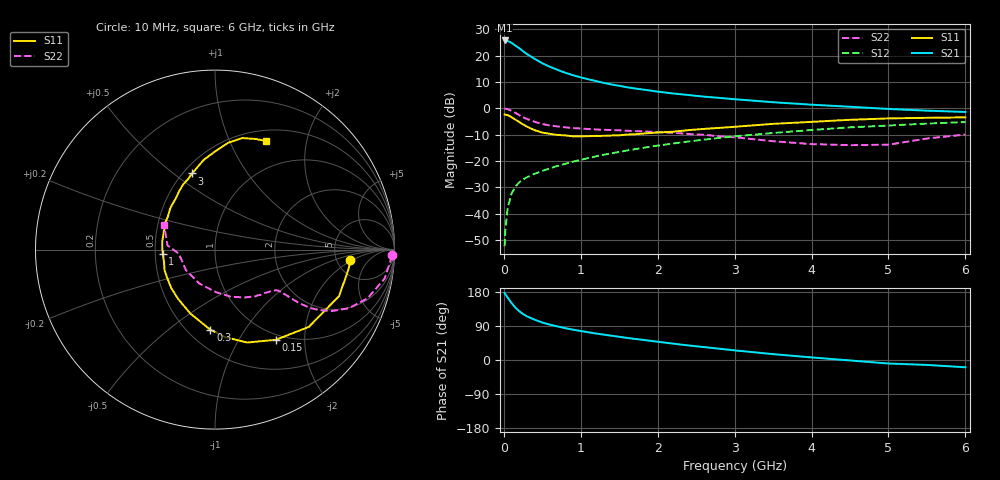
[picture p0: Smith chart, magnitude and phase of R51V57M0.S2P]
! SIEMENS Small Signal Semiconductors
! BFR183
! Si NPN RF Bipolar Junction Transistor in SOT23
! VCE = 1.5 V  IC = 7 mA
! Common Emitter S-Parameters:  May  1996
# GHz  S  MA  R  50
!  f  S11  S21  S12  S22
! GHz  MAG  ANG  MAG  ANG  MAG  ANG  MAG  ANG
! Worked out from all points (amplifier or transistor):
!   36 points, 10 MHz to 6 GHz, reference 50 ohm
!   highest |S21| = 25.7 dB at 10 MHz (marker M1)
!   |S21| within 3 dB of that: start of sweep to 202.1 MHz
!   unconditionally stable (mu >= 1): 860 MHz to 2.635 GHz
!   at 250 MHz: K = 0.52, MSG = 24.4 dB, |S12| = -27.1 dB
!   at 1.4 GHz: K = 1.07, MAG = 11.5 dB, |S12| = -17.1 dB
!   at 6 GHz: K = 0.91, MSG = 1.9 dB, |S12| = -5.3 dB
!   S11 on the Smith chart (normalised r, x): 10 MHz: 6.73, -1.78; 150 MHz: 0.92, -1.46; 300 MHz: 0.64, -0.71; 1 GHz: 0.55, -0.03; 3 GHz: 0.55, +0.59; 6 GHz: 0.63, +1.38
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0.01  0.7564 -4.3  19.3 177.0  0.0024 87.6  0.9845 -1.9
0.02  0.7521 -8.4  19.07 173.5  0.005 81.4  0.9788 -3.9
0.05  0.738 -20.6  18.85 164.4  0.0128 80.2  0.9589 -9.7
0.1  0.6772 -39.5  17.44 150.4  0.0239 72.3  0.8914 -17.8
0.15  0.6062 -56.0  15.43 138.2  0.0324 65.9  0.8135 -23.7
0.2  0.5479 -70.9  13.74 128.8  0.0391 62.3  0.7382 -27.6
0.25  0.492 -83.0  12.06 121.2  0.0442 59.8  0.672 -30.1
0.3  0.4475 -93.3  10.66 115.3  0.0489 58.3  0.6234 -31.5
0.4  0.3815 -111.2  8.633 106.3  0.0569 57.4  0.5513 -32.5
0.5  0.3442 -126.1  7.132 98.9  0.0643 58.2  0.5001 -32.6
0.6  0.3256 -138.2  6.093 93.3  0.0724 58.7  0.47 -32.6
0.7  0.31 -148.9  5.32 88.4  0.0802 59.6  0.4493 -32.7
0.8  0.3041 -157.6  4.696 84.0  0.0879 59.8  0.4328 -32.8
1  0.2924 -175.5  3.841 76.5  0.1044 60.9  0.4104 -33.5
1.1  0.2941 177.8  3.537 73.2  0.1132 61.0  0.402 -34.5
1.6  0.3156 150.6  2.497 58.3  0.1571 59.7  0.3726 -40.1
2.2  0.3573 128.1  1.9 43.2  0.2134 55.8  0.3412 -50.3
3  0.4433 106.7  1.479 25.4  0.2922 47.8  0.2805 -70.5
3.5  0.5037 97.2  1.298 15.5  0.3381 41.7  0.236 -89.3
4.5  0.6014 82.7  1.064 -1.2  0.4329 29.2  0.1985 -144.6
5.5  0.6564 69.9  0.897 -13.0  0.51 17.0  0.2657 174.9
6  0.6695 64.7  0.847 -19.2  0.5446 9.1  0.3156 154.0
